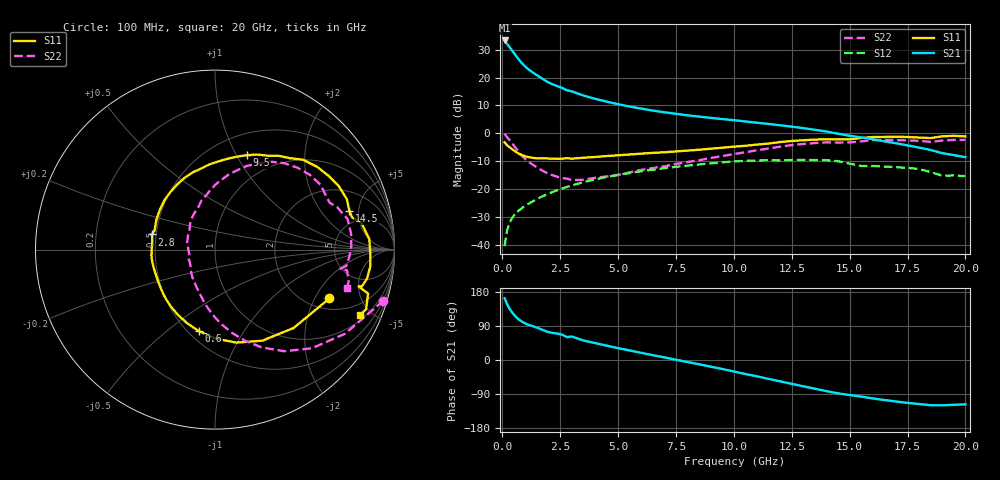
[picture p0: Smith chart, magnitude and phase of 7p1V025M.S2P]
! Infineon Technologies  Discrete & RF Semiconductors
! bfp620
! VCE =  1.0 V,  IC =  25 mA
! Common Emitter S-Parameters:  Sep 2002
# GHz  S  MA  R  50
!  f  S11  S21  S12  S22
! GHz  MAG  ANG  MAG  ANG  MAG  ANG  MAG  ANG
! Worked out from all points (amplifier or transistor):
!   59 points, 100 MHz to 20 GHz, reference 50 ohm
!   highest |S21| = 33.3 dB at 100 MHz (marker M1)
!   |S21| within 3 dB of that: start of sweep to 371.5 MHz
!   unconditionally stable (mu >= 1): 3.274 GHz to 9.969 GHz; 17.12 GHz to end of sweep
!   at 1 GHz: K = 0.74, MSG = 24.9 dB, |S12| = -25.9 dB
!   at 5.5 GHz: K = 1.04, MAG = 10.7 dB, |S12| = -14.2 dB
!   at 20 GHz: K = 1.39, MAG = -0.3 dB, |S12| = -15.3 dB
!   S11 on the Smith chart (normalised r, x): 100 MHz: 2.53, -2.65; 600 MHz: 0.56, -0.65; 2.8 GHz: 0.47, +0.09; 9.5 GHz: 0.73, +1.10; 14.5 GHz: 3.58, +3.92; 20 GHz: 1.26, -4.27
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0.1  0.6932 -23.1  46.1 163.0  0.0096 84.5  0.9801 -16.9
0.2  0.6185 -44.9  40.25 148.2  0.0178 71.2  0.8631 -32.9
0.3  0.572 -62.5  35.65 136.5  0.0243 65.4  0.7707 -45.5
0.4  0.532 -77.0  31.5 127.3  0.0295 61.8  0.6854 -55.7
0.5  0.4954 -89.7  27.71 119.7  0.0339 59.3  0.6056 -64.3
0.6  0.4637 -101.0  24.32 113.3  0.0377 57.5  0.5338 -71.9
0.7  0.4379 -111.1  21.43 107.8  0.0412 56.3  0.472 -78.6
0.8  0.4178 -119.8  19.03 103.2  0.0445 55.5  0.4208 -84.6
0.9  0.4022 -127.3  17.11 99.4  0.0477 55.0  0.3794 -89.8
1.2  0.3722 -143.8  13.34 91.6  0.0572 54.2  0.2971 -101.9
1.9  0.356 -171.0  8.616 75.7  0.0803 51.5  0.199 -129.1
2.8  0.3618 166.5  5.909 60.3  0.1106 45.5  0.1552 -161.2
3  0.3532 162.6  5.665 62.1  0.1173 43.9  0.1455 -163.7
3.5  0.3668 152.9  4.776 51.5  0.134 39.6  0.1485 -179.4
5  0.4059 127.6  3.336 31.3  0.1813 25.6  0.1806 141.7
7  0.4595 99.2  2.388 6.9  0.2388 6.1  0.2572 110.6
9.5  0.5551 71.4  1.807 -23.7  0.3038 -20.8  0.3931 84.3
10.5  0.6005 60.5  1.636 -37.0  0.3232 -33.4  0.4604 74.2
13.5  0.7753 27.0  1.163 -75.7  0.3335 -69.0  0.6729 38.3
14.5  0.7787 16.1  0.988 -88.0  0.3182 -84.2  0.6867 25.9
17  0.8703 -6.1  0.667 -109.5  0.249 -100.2  0.7599 1.6
20  0.8859 -24.4  0.376 -117.1  0.1719 -110.8  0.7661 -16.0
